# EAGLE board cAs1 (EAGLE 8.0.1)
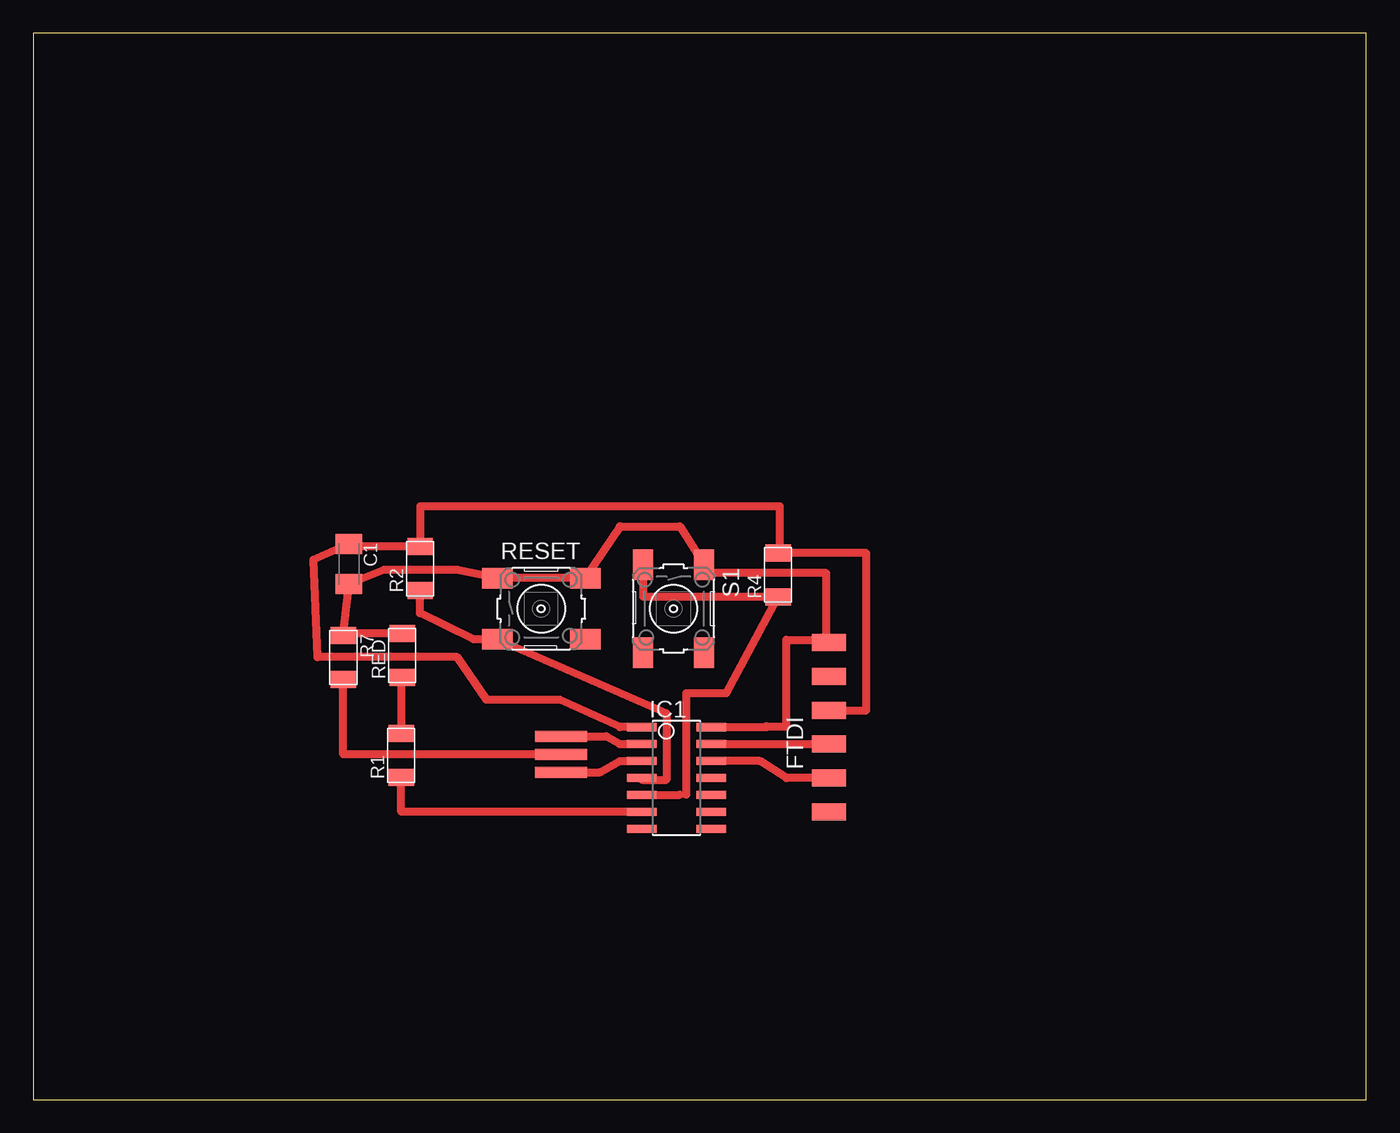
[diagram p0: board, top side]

Size 100 x 80 mm. Coordinates in mm from the lower left corner, seen from the top.
Outline: 0,0 100,0 100,80 0,80 0,0
Copper layers (1*16): Top 0.035mm / dielectric 1.5mm / Bottom 0.035mm
Design rules "default": minimum track width 10mil, minimum drill 24mil, track to track 8mil, track to pad 8mil, pad to pad 8mil, via to via 8mil, smd to smd 8mil, copper to edge 40mil, drill to drill 8mil, minimum pad ring 10mil, minimum via ring 8mil, stop-mask expansion 4mil, vias tented up to drill 0mil, thermal gap 10mil

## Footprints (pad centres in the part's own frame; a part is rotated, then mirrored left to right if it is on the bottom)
EFOBM = smd 0.8 x 3.9: 1 -1.35,0; 2 0,0; 3 1.35,0
C1206K = smd 1.5 x 2: 1 -1.5,0; 2 1.5,0
1X06SMD = smd 2.54 x 1.27: 1 0,6.35; 2 0,3.81; 3 0,1.27; 4 0,-1.27; 5 0,-3.81; 6 0,-6.35
SOIC14 = smd 0.61 x 2.21: 1 -3.81,-2.603; 2 -2.54,-2.603; 3 -1.27,-2.603; 4 0,-2.603; 5 1.27,-2.603; 6 2.54,-2.603; 7 3.81,-2.603; 8 3.81,2.603; 9 2.54,2.603; 10 1.27,2.603; 11 0,2.603; 12 -1.27,2.603; 13 -2.54,2.603; 14 -3.81,2.603
R1206FAB = smd 1.27 x 1.905: 1 -1.651,0; 2 1.651,0
LED1206FAB = smd 1.27 x 1.905: 1 -1.651,0; 2 1.651,0
6MM_SWITCH = smd 2.286 x 1.524: 1 -3.302,2.286; 2 3.302,2.286; 3 -3.302,-2.286; 4 3.302,-2.286

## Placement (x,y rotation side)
20MHZ  RESONATOR  [EFOBM]  39.6,25.9 270 top
C1  0.1uF  [C1206K]  23.68,40.18 270 top
FTDI  FTDI-SMD-HEADER  [1X06SMD]  59.69,27.94 0 top
IC1  ATTINY44-SSU  [SOIC14]  48.26,24.13 270 top
R1  499R  [R1206FAB]  27.6,25.83 90 top
R2  4.99k  [R1206FAB]  29.02,39.83 90 top
R4  4.99K  [R1206FAB]  55.88,39.37 90 top
R7  0  [R1206FAB]  23.26,33.18 270 top
RED  LEDFAB1206  [LED1206FAB]  27.68,33.33 90 top
RESET  [6MM_SWITCH]  38.1,36.83 0 top
S1  [6MM_SWITCH]  48.03,36.83 270 top

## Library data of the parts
20MHZ C1 FTDI IC1 R1 R2 R4 R7 RED RESET S1 = fab

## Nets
GND: C1.2 FTDI.1 IC1.14 R7.1 RED.2 RESET.1 RESET.2 S1.1
MISO: IC1.8
MOSI: IC1.7
N$1: R1.2 RED.1
N$2: 20MHZ.2 R7.2
PA2: IC1.11
PA3: IC1.10
PA7: IC1.6 R1.1
PB2: IC1.5 R4.1 S1.3
RST: IC1.4 R2.1 RESET.3
RX: FTDI.5 IC1.12
SCK: IC1.9
TX: FTDI.4 IC1.13
VCC: C1.1 FTDI.3 IC1.1 R2.2 R4.2
X1: 20MHZ.1 IC1.2
X2: 20MHZ.3 IC1.3

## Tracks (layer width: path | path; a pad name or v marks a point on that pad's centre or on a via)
GND
  Top 0.61: IC1.14 55,27.94 55,28 56.5,28 56.5,34.5 59.69,34.5 FTDI.1 59.5,34.29 59.5,39.5 50.32,39.5 S1.1 48.5,43 44,43 RESET.2 RESET.1 | RESET.1 34.8,39.5 | RED.2 23.26,34.98 R7.1 C1.2 26.3,39.75 31.8,39.75 RESET.1
N$1
  Top 0.61: RED.1 27.6,31.68 R1.2
N$2
  Top 0.61: 20MHZ.2 23.26,25.9 R7.2
PA7
  Top 0.61: IC1.6 27.6,21.59 R1.1
PB2
  Top 0.406: 48.5,22.86 49,22.86
  Top 0.61: IC1.5 48.5,22.86 | 45.74,39.5 S1.3 45.74,37.72 R4.1 52,30.5 49,30.5 49,22.86
RST
  Top 0.61: R2.1 29,38.18 29,36.5 33,34.54 RESET.3 | RESET.3 35,34.54 | IC1.4 45.66,24 47.5,24 47.5,29 RESET.3
RX
  Top 0.61: IC1.12 54.5,25.4 56.5,24.13 FTDI.5
TX
  Top 0.61: IC1.13 FTDI.4
VCC
  Top 0.61: IC1.1 44,27.94 39.5,30 34,30 31.8,33.2 21.3,33.2 21,40.5 C1.1 23.68,41.48 R2.2 29.02,44.5 56,44.5 56,41.02 R4.2 55.88,41 62.5,41 62.5,29.21 FTDI.3
X1
  Top 0.61: 20MHZ.1 43,27.25 44,26.67 IC1.2
X2
  Top 0.61: 20MHZ.3 42.5,24.55 44,25.4 IC1.3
